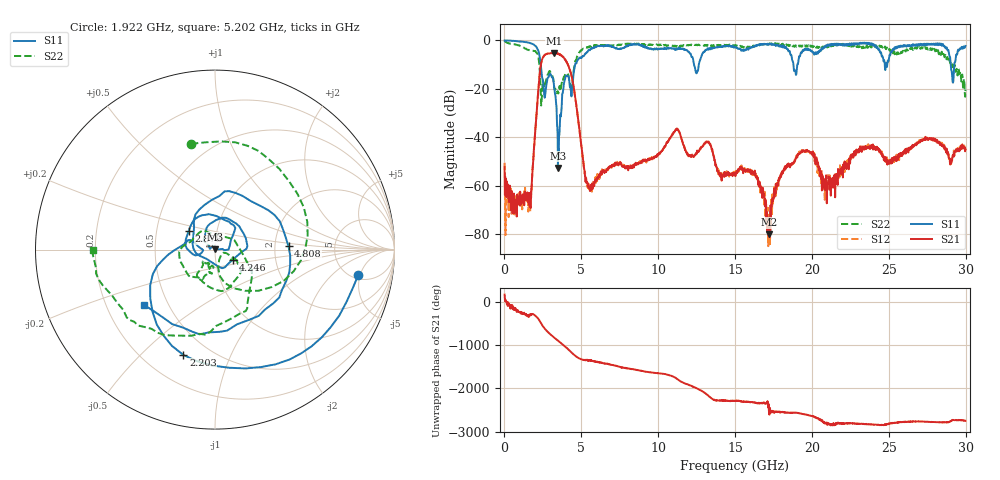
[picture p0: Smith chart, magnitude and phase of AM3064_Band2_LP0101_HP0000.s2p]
# Hz S DB R 50.0
!freq dBS11 angS11 dBS21 angS21 dBS12 angS12 dBS22 angS22
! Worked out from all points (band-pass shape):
!   1600 points, 10 MHz to 29.98 GHz, reference 50 ohm
!   highest |S21| = -5.17 dB at 3.234 GHz (marker M1); lowest = -80.0 dB at 17.2 GHz (marker M2)
!   |S21| within 3 dB of the highest: 2.434 GHz to 3.964 GHz (1.531 GHz wide, 47.8 % of centre)
!   lowest |S11| = -52.7 dB at 3.478 GHz (marker M3), VSWR 1.00, Z = 50.2 + j0.167 ohm
!   |S11| at or under -10 dB: 2.362 GHz to 4.594 GHz (2.233 GHz wide, 64.2 % of centre); 12.33 GHz to 12.64 GHz (312.8 MHz wide, 2.51 % of centre); 18.8 GHz to 19.05 GHz (250.6 MHz wide, 1.32 % of centre)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
!   |S22| runs from -26.9 to -0.2 dB; largest |S21 - S12| = 0.016
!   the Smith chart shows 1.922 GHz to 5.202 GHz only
!   S11 on the Smith chart (normalised r, x): 1.922 GHz: 5.65, -4.66; 2.203 GHz: 0.36, -0.68; 2.878 GHz: 0.73, +0.16; 4.246 GHz: 1.21, -0.14; 4.808 GHz: 2.38, +0.11; 5.202 GHz: 0.37, -0.30
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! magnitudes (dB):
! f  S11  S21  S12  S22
! 10 MHz  0.0  -52.3  -50.5  -0.2
! 1.584 GHz  -1.0  -67.3  -63.5  -4.0
! 1.922 GHz  -1.8  -44.2  -44.8  -4.4
! 2.203 GHz  -4.3  -20.6  -20.5  -6.8
! 2.878 GHz  -14.9  -5.4  -5.4  -13.2
! 3.234 GHz  -19.5  -5.2  -5.1  -19.4
! 3.478 GHz  -52.7  -5.5  -5.6  -21.3
! 4.246 GHz  -18.8  -12.0  -12.0  -17.8
! 4.808 GHz  -7.7  -33.3  -33.2  -5.6
! 5.015 GHz  -7.3  -44.3  -44.0  -4.2
! 5.202 GHz  -6.0  -54.0  -53.4  -3.4
! 10 GHz  -3.5  -47.0  -46.8  -1.9
! 11.22 GHz  -3.8  -36.3  -36.5  -2.3
! 15 GHz  -2.6  -55.5  -55.1  -1.9
! 16.34 GHz  -2.4  -56.2  -54.4  -2.4
! 17.2 GHz  -1.5  -80.0  -82.7  -1.6
! 18.17 GHz  -2.6  -53.6  -53.5  -2.2
! 19.99 GHz  -4.3  -47.1  -47.0  -2.2
! 20.93 GHz  -2.2  -55.6  -59.9  -2.2
! 23.21 GHz  -1.4  -44.9  -45.0  -2.4
! 25 GHz  -8.0  -50.5  -50.0  -3.3
! 29.98 GHz  -2.3  -45.0  -44.7  -20.3
